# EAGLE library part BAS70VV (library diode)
Silicon Schottky Diodes General-purpose diode for high-speed switching Source: BAS70_1PS7XSB70_SER_8.pdf
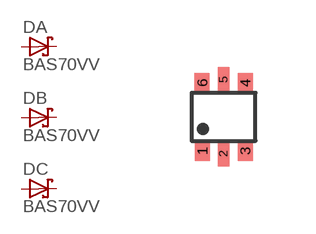
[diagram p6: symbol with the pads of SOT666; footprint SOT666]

Designator prefix D; gates A=SCHOTTKY B=SCHOTTKY C=SCHOTTKY

## BAS70VV  [SOT666]
1  A:A  pas
2  B:A  pas
3  C:A  pas
4  C:C  pas
5  B:C  pas
6  A:C  pas

## Footprint SOT666 (pad centres in mm)
SOT 666 Reflow soldering foorprint Source: Philips - BAS70_1PS7XSB70_SER_8.pdf
smd 0.375 x 0.5: 1 -0.537,-0.85; 3 0.538,-0.85; 4 0.538,0.849; 6 -0.538,0.85
smd 0.3 x 0.65: 2 0,-0.923; 5 0,0.925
